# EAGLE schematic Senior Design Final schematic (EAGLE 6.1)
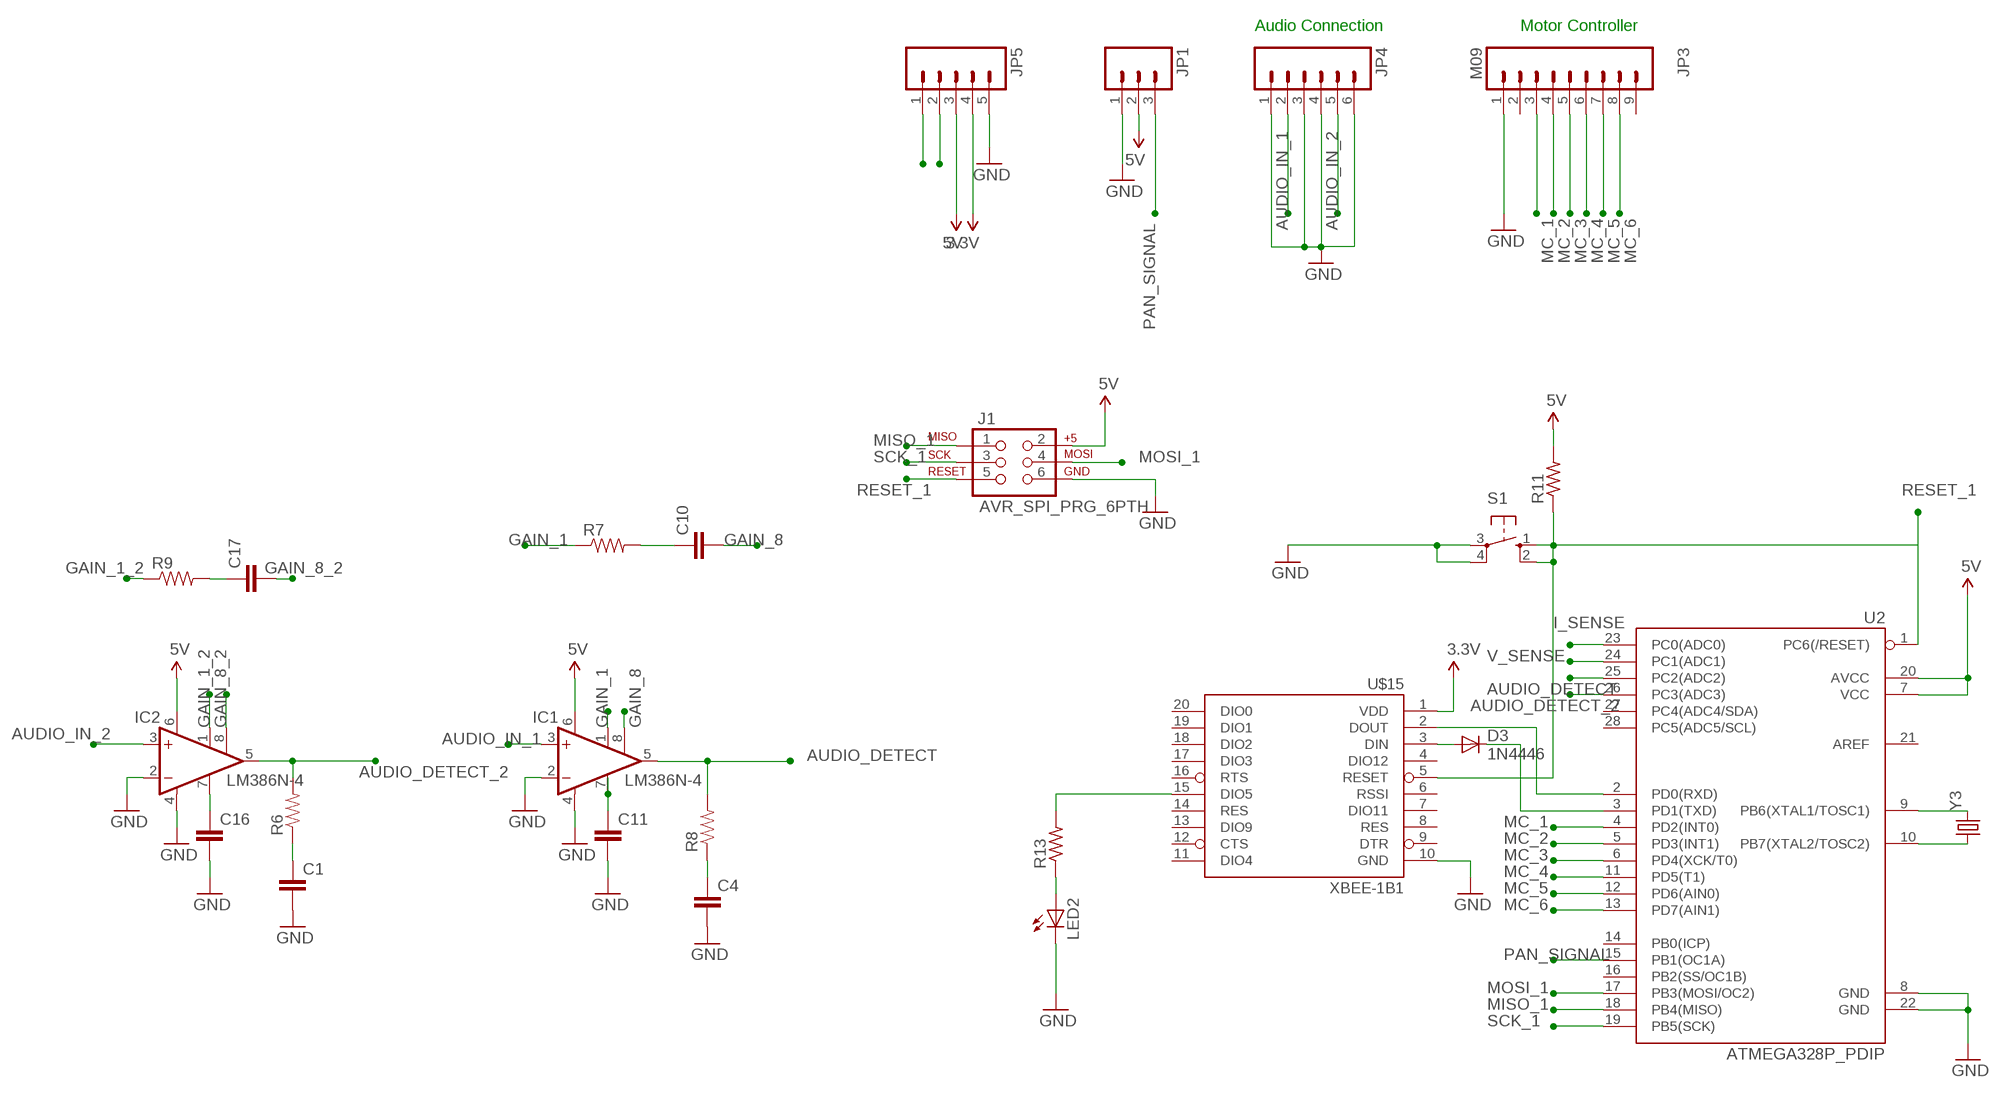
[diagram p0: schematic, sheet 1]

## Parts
C1  CAPPTH1  [CAP-PTH-5MM]
C4  CAPPTH1  [CAP-PTH-5MM]
C10  CAPPTH3  [CAP-PTH-LARGE]
C11  CAPPTH1  [CAP-PTH-5MM]
C16  CAPPTH1  [CAP-PTH-5MM]
C17  CAPPTH3  [CAP-PTH-LARGE]
D3  1N4446  [DO35-10]
IC1  LM386N-4  [DIL08]
IC2  LM386N-4  [DIL08]
J1  AVR_SPI_PRG_6PTH  [2X3]
JP1  M03PTH  [1X03]
JP3  M09  [1X09]
JP4  M06SIP  [1X06]
JP5  M05PTH  [1X05]
LED2  LED5MM  [LED5MM]
R6  RESISTORAXIAL-0.3  [AXIAL-0.3]
R7  RESISTORAXIAL-0.3  [AXIAL-0.3]
R8  RESISTORAXIAL-0.3  [AXIAL-0.3]
R9  RESISTORAXIAL-0.3  [AXIAL-0.3]
R11  R-US_0207/10  [0207/10]
R13  R-US_0207/10  [0207/10]
S1  40-XX  [B3F-40XX]
U2  ATMEGA328P_PDIP  [DIL28-3]
U$15  XBEE-1B1  [XBEE-1]
Y3  CRYSTALHC49US  [HC49US]

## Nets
3.3V: JP5.4 U$15.1(VDD)
5V: IC1.6(VS) IC2.6(VS) J1.2 JP1.2 JP5.3 R11.2 U2.7(VCC) U2.20(AVCC)
AUDIO_DETECT: IC1.5(OUT) R8.P$2 U2.25(PC2(ADC2))
AUDIO_DETECT_2: IC2.5(OUT) R6.P$2 U2.26(PC3(ADC3))
AUDIO_IN_1: IC1.3(+IN) JP4.2
AUDIO_IN_2: IC2.3(+IN) JP4.5
GAIN_1: IC1.1(GAIN) R7.P$1
GAIN_1_2: IC2.1(GAIN) R9.P$1
GAIN_8: C10.2 IC1.8(GAIN)
GAIN_8_2: C17.2 IC2.8(GAIN)
GND: C1.2 C4.2 C11.2 C16.2 IC1.2(-IN) IC1.4(GND) IC2.2(-IN) IC2.4(GND) J1.6 JP1.1 JP3.1 JP4.1 JP4.3 JP4.4 JP4.6 JP5.5 LED2.K(C) S1.3(P) S1.4(P1) U2.8(GND) U2.22(GND) U$15.10(GND)
I_SENSE: JP5.2 U2.23(PC0(ADC0))
MC_1: JP3.3 U2.4(PD2(INT0))
MC_2: JP3.4 U2.5(PD3(INT1))
MC_3: JP3.5 U2.6(PD4(XCK/T0))
MC_4: JP3.6 U2.11(PD5(T1))
MC_5: JP3.7 U2.12(PD6(AIN0))
MC_6: JP3.8 U2.13(PD7(AIN1))
MISO_1: J1.1 U2.18(PB4(MISO))
MOSI_1: J1.4 U2.17(PB3(MOSI/OC2))
N$1: R13.2 U$15.15(DIO5)
N$2: D3.C U2.3(PD1(TXD))
N$3: D3.A U$15.3(DIN)
N$4: U2.2(PD0(RXD)) U$15.2(DOUT)
N$12: C11.1 IC1.7(BYPASS)
N$13: C10.1 R7.P$2
N$16: U2.10(PB7(XTAL2/TOSC2)) Y3.1
N$17: U2.9(PB6(XTAL1/TOSC1)) Y3.2
N$20: LED2.A R13.1
N$24: C16.1 IC2.7(BYPASS)
N$27: C1.1 R6.P$1
N$28: C4.1 R8.P$1
N$29: C17.1 R9.P$2
PAN_SIGNAL: JP1.3 U2.15(PB1(OC1A))
RESET_1: J1.5 R11.1 S1.1(S) S1.2(S1) U2.1(PC6(/RESET)) U$15.5(RESET)
SCK_1: J1.3 U2.19(PB5(SCK))
V_SENSE: JP5.1 U2.24(PC1(ADC1))
Unconnected: JP3.2 JP3.9 U2.14(PB0(ICP)) U2.16(PB2(SS/OC1B)) U2.21(AREF) U2.27(PC4(ADC4/SDA)) U2.28(PC5(ADC5/SCL)) U$15.4(DIO12) U$15.6(RSSI) U$15.7(DIO11) U$15.8(RES) U$15.9(DTR) U$15.11(DIO4) U$15.12(CTS) U$15.13(DIO9) U$15.14(RES) U$15.16(RTS) U$15.17(DIO3) U$15.18(DIO2) U$15.19(DIO1) U$15.20(DIO0)

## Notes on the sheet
- Audio Connection | Motor Controller

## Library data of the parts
C1 C4 C10 C11 C16 C17 = SparkFun-Passives:CAP: Capacitor
D3 = diode:1N4446: DIODE
IC1 IC2 = linear:LM386?-*: Low Voltage Audio Power Amplifier Source: http://cache.national.com/ds/LM/LM386.pdf
J1 = SparkFun-Connectors:AVR_SPI_PRG_6: AVR ISP 6 Pin This is the reduced ISP connector for AVR programming. Common on Arduino. This footprint will take up less PCB space and can be used with a 10-pin to 6-pin adapter such as SKU: BOB-08508
JP1 = SparkFun-Connectors:M03: Header 3 Standard 3-pin 0.1" header. Use with straight break away headers (SKU : PRT-00116), right angle break away headers (PRT-00553), swiss pins (PRT-00743), machine pins (PRT-00117), and female headers (PRT-00115). Molex polarized connector foot print use with SKU : PRT-08232 with associated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
JP3 = SparkFun-Connectors:M09: Header 9 Standard 9-pin 0.1" header. Use with straight break away headers (SKU : PRT-00116), right angle break away headers (PRT-00553), swiss pins (PRT-00743), machine pins (PRT-00117), and female headers (PRT-00115).
JP4 = SparkFun-Connectors:M06: Header 6 Standard 6-pin 0.1" header. Use with straight break away headers (SKU : PRT-00116), right angle break away headers (PRT-00553), swiss pins (PRT-00743), machine pins (PRT-00117), and female headers (PRT-00115). Molex polarized connector foot print use with SKU : PRT-08094 with associated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
JP5 = SparkFun-Connectors:M05: Header 5 Standard 5-pin 0.1" header. Use with straight break away headers (SKU : PRT-00116), right angle break away headers (PRT-00553), swiss pins (PRT-00743), machine pins (PRT-00117), and female headers (PRT-00115). Molex polarized connector foot print use with SKU : PRT-08230 with associated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
LED2 = SparkFun-LED:LED: LEDs
R6-R9 = SparkFun-Passives:RESISTOR: Resistor
R11 R13 = rcl:R-US_: RESISTOR, American symbol
S1 = switch-omron:40-XX: OMRON SWITCH; MF: OMRON COMPONENTS USA; MPN: B3F-4000; OC_FARNELL: 176434; OC_NEWARK: 36K3105
U2 = SparkFun-DigitalIC:ATMEGA328P_PDIP: uC used in the Arduino 32kb flash, 1k EEPROM, 2k SRAM This is the through-hole version of this chip.
U$15 = SparkFun-RF:XBEE-1: Xbee module footprints
Y3 = SparkFun-FreqCtrl:CRYSTAL: Various standard crystals. Proven footprints. Spark Fun Electronics SKU : COM-00534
